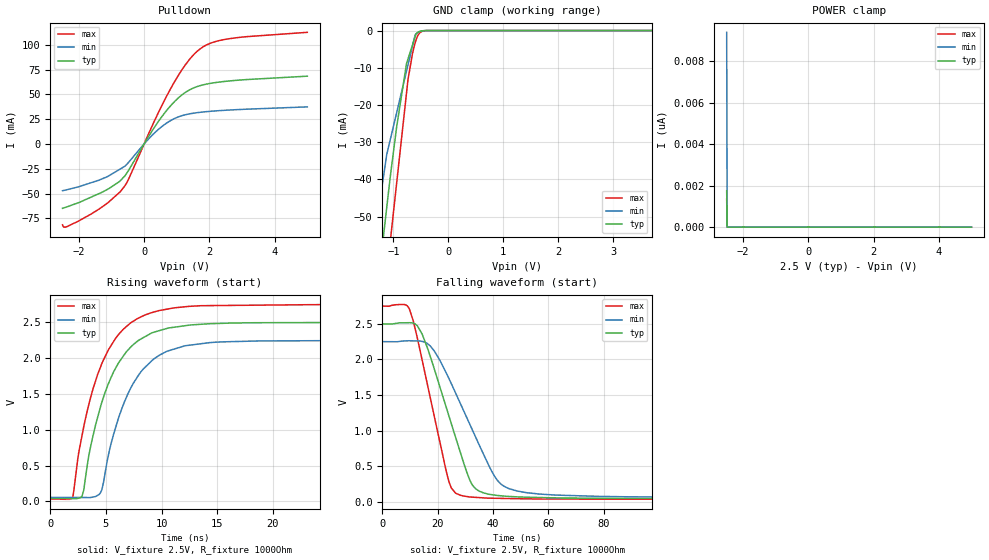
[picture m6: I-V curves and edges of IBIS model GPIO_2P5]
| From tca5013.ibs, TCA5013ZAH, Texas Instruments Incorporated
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[Model]   GPIO_2P5
Model_type   I/O_open_drain
Polarity   Non-Inverting
Enable   Active-Low
Vinl = .4
Vinh = 1.4
Vmeas = 1.25
Vref = 2.5
Cref = 15pF
Rref = 1000
|   typ   min   max
C_comp   1.055p   0.761p   1.480p
|C_comp (Low state)   1.233p   0.829p   1.541p
|C_comp (High state)   1.055p   0.761p   1.480p
[Voltage Range]   2.5   2.25   2.75
[Temperature Range]   27   125   -40
[Pullup Reference]   2.5   2.25   2.75
[Pulldown Reference]   0   0   0
[Power Clamp Reference]   2.5   2.25   2.75
[GND Clamp Reference]   0   0   0
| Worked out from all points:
|   slope of the pulldown table from 0 to 0.375 V, typ, clamps not added: 19.1 ohm
|   GND clamp passes 1 mA (typ) near -0.59 V on its own axis
|   falling waveform, V_fixture 2.5V, R_fixture 1000Ohm: 20-80 % time 11.9ns typ, 15.6ns min, 9.07ns max; typ from 2.5 V to 0.042 V
|   rising waveform, V_fixture 2.5V, R_fixture 1000Ohm: 20-80 % time 3.12ns typ, 3.12ns min, 3.13ns max; typ from 0.042 V to 2.5 V
[Pulldown]
|   Voltage   I(typ)   I(min)   I(max)
-2.5V     -64.91mA   -47.2mA    -81.59mA
-2.41V    -63.98mA   -46.55mA   -83.94mA
-1.615V   -53.53mA   -39.04mA   -70.55mA
-1.12V    -45.76mA   -32.91mA   -59.63mA
-587.5mV  -32.21mA   -22.47mA   -42.16mA
215mV     11.64mA    7.735mA    15.96mA
740mV     35.76mA    22.14mA    51.34mA
1.235V    51.32mA    29.19mA    78.45mA
1.685V    58.48mA    31.77mA    95.09mA
2.03V     61.09mA    32.9mA     101.5mA
2.525V    63.23mA    34.02mA    105.7mA
5V        68.33mA    37.36mA    112.6mA
[GND Clamp]
|   Voltage   I(typ)   I(min)   I(max)
-2.5V     -248mA     -195.5mA   -300.9mA
-1.345V   -77.34mA   -56.02mA   -101.5mA
-1.3V     -71.05mA   -51.26mA   -94.09mA
-1.12V    -47.53mA   -33.31mA   -65.32mA
-1.045V   -38.01mA   -28.64mA   -55.2mA
-940mV    -25.91mA   -22.1mA    -41.03mA
-760mV    -8.866mA   -10.89mA   -16.74mA
-735.6mV  -7.744mA   -9.367mA   -13.45mA
-603.6mV  -1.663mA   -1.142mA   -3.334mA
-535mV    -315.2uA   -398.2uA   -920.3uA
-355mV    -2.921uA   -10.24uA   -4.448uA
5V        0A         0A         0A
[POWER Clamp]
|   Voltage   I(typ)   I(min)   I(max)
-2.5V     1.746nA    9.39nA     1.348nA
-2.485V   0A         0A         0A
-2.478V   0A         0A         0A
5V        0A         0A         0A
[Ramp]
R_load = 1000
|   typ   min   max
dV/dt_r   1.47505/3.09184e-09   1.31632/3.12045e-09   1.63008/3.10467e-09
dV/dt_f   1.47495/1.18882e-08   1.31596/1.5576e-08   1.63006/9.07359e-09
[Falling Waveform]
V_fixture = 2.5V
V_fixture_min = 2.25V
V_fixture_max = 2.75V
R_fixture = 1000Ohm
C_fixture = 0F
|   Time   V(typ)   V(min)   V(max)
0s        2.5V       2.25V      2.75V
9.738ns   2.516V     2.262V     2.711V
14.37ns   2.358V     2.253V     1.992V
18.83ns   1.858V     2.115V     1.188V
23.68ns   1.252V     1.762V     336.1mV
28.17ns   695.2mV    1.382V     90.65mV
33.66ns   183mV      911.5mV    60.92mV
41.48ns   87.91mV    304.9mV    47.51mV
48.66ns   68.06mV    150.2mV    42.18mV
199.9ns   41.75mV    56.74mV    33.23mV
[Rising Waveform]
V_fixture = 2.5V
V_fixture_min = 2.25V
V_fixture_max = 2.75V
R_fixture = 1000Ohm
C_fixture = 0F
|   Time   V(typ)   V(min)   V(max)
0s        41.59mV    56.13mV    33.2mV
2.036ns   39.08mV    55.27mV    68.04mV
2.855ns   74.07mV    54.92mV    920.6mV
3.629ns   768mV      55.34mV    1.453V
4.629ns   1.381V     159.2mV    1.923V
5.855ns   1.856V     1.022V     2.274V
6.96ns    2.11V      1.496V     2.458V
8.33ns    2.284V     1.844V     2.59V
12.41ns   2.46V      2.18V      2.723V
199.9ns   2.5V       2.25V      2.75V
